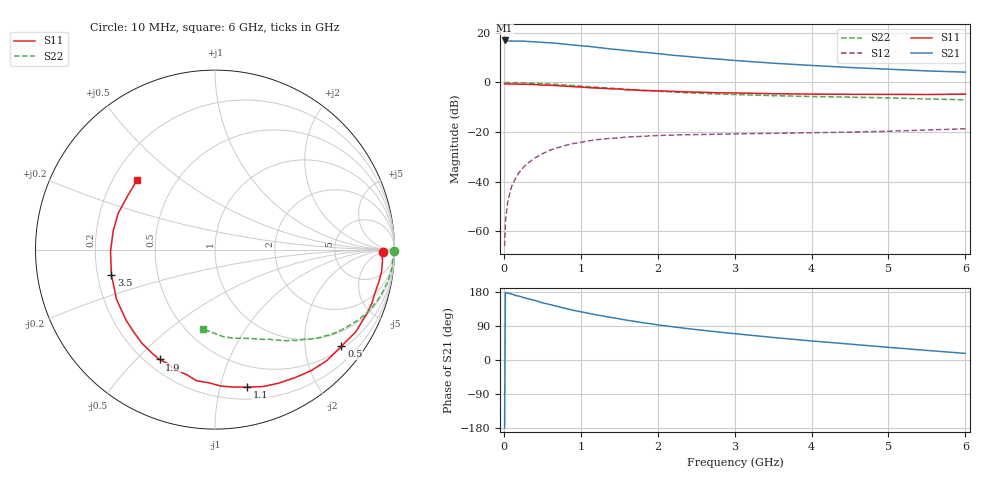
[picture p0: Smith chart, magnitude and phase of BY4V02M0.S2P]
! SIEMENS Small Signal Semiconductors
! BFY420
! Si NPN RF SIEGET Grounded Emitter Transistor in MICRO-X
! VCE = 4 V  IC = 2 mA
! Common Emitter S-Parameters:  October  1996
# GHz  S  MA  R  50
!  f  S11  S21  S12  S22
! GHz  MAG  ANG  MAG  ANG  MAG  ANG  MAG  ANG
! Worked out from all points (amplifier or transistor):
!   36 points, 10 MHz to 6 GHz, reference 50 ohm
!   highest |S21| = 16.9 dB at 10 MHz (marker M1)
!   |S21| within 3 dB of that: start of sweep to 1.272 GHz
!   unconditionally stable (mu >= 1): 3.993 GHz to end of sweep
!   at 250 MHz: K = 0.08, MSG = 25.5 dB, |S12| = -34.4 dB
!   at 1.4 GHz: K = 0.29, MSG = 18.0 dB, |S12| = -22.6 dB
!   at 6 GHz: K = 1.24, MAG = 8.5 dB, |S12| = -18.7 dB
!   S11 on the Smith chart (normalised r, x): 10 MHz: 28, -6; 500 MHz: 0.57, -2.85; 1.1 GHz: 0.30, -1.22; 1.9 GHz: 0.25, -0.59; 3.5 GHz: 0.26, -0.11; 6 GHz: 0.30, +0.35
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0.01  0.934 -0.8  7.033 -179.7  0.0005 51.4  0.9962 -0.4
0.02  0.93 -1.6  6.983 178.4  0.0015 71.2  0.9934 -0.7
0.05  0.9357 -3.9  6.843 176.5  0.0039 77.4  0.9948 -1.7
0.1  0.9359 -7.8  6.875 174.5  0.008 81.6  0.9911 -3.5
0.15  0.9304 -11.2  6.813 170.5  0.0114 80.3  0.991 -5.4
0.2  0.9234 -15.3  6.809 168.4  0.0154 80.2  0.989 -7.0
0.25  0.924 -19.0  6.823 165.2  0.0191 77.3  0.9837 -8.8
0.4  0.9083 -30.3  6.595 157.4  0.0298 72.1  0.9649 -13.9
0.5  0.8865 -37.4  6.432 151.0  0.0365 68.2  0.95 -17.1
0.6  0.8778 -44.8  6.317 146.3  0.0432 64.6  0.9322 -20.3
0.8  0.8413 -58.0  5.901 136.2  0.0539 56.9  0.8894 -26.1
0.9  0.8242 -64.6  5.682 131.4  0.0585 53.8  0.8678 -28.6
1.1  0.7869 -76.8  5.35 123.2  0.0662 48.6  0.8254 -33.6
1.4  0.7427 -92.7  4.707 112.0  0.0743 41.3  0.7653 -39.7
1.6  0.7129 -103.2  4.382 104.9  0.0793 37.2  0.7268 -43.3
1.9  0.6857 -116.8  3.964 95.9  0.0837 32.2  0.6812 -48.0
2.2  0.6616 -128.1  3.535 87.6  0.087 28.3  0.6444 -52.0
2.8  0.62 -147.6  2.951 73.6  0.0907 23.3  0.582 -59.1
3.5  0.5936 -166.4  2.449 59.5  0.0944 20.0  0.5421 -66.4
4.5  0.5768 169.8  2.003 41.9  0.0997 18.0  0.5059 -77.5
5.5  0.5717 148.0  1.71 25.3  0.11 17.6  0.465 -90.9
6  0.5822 138.0  1.613 17.4  0.1164 16.9  0.4474 -98.7
